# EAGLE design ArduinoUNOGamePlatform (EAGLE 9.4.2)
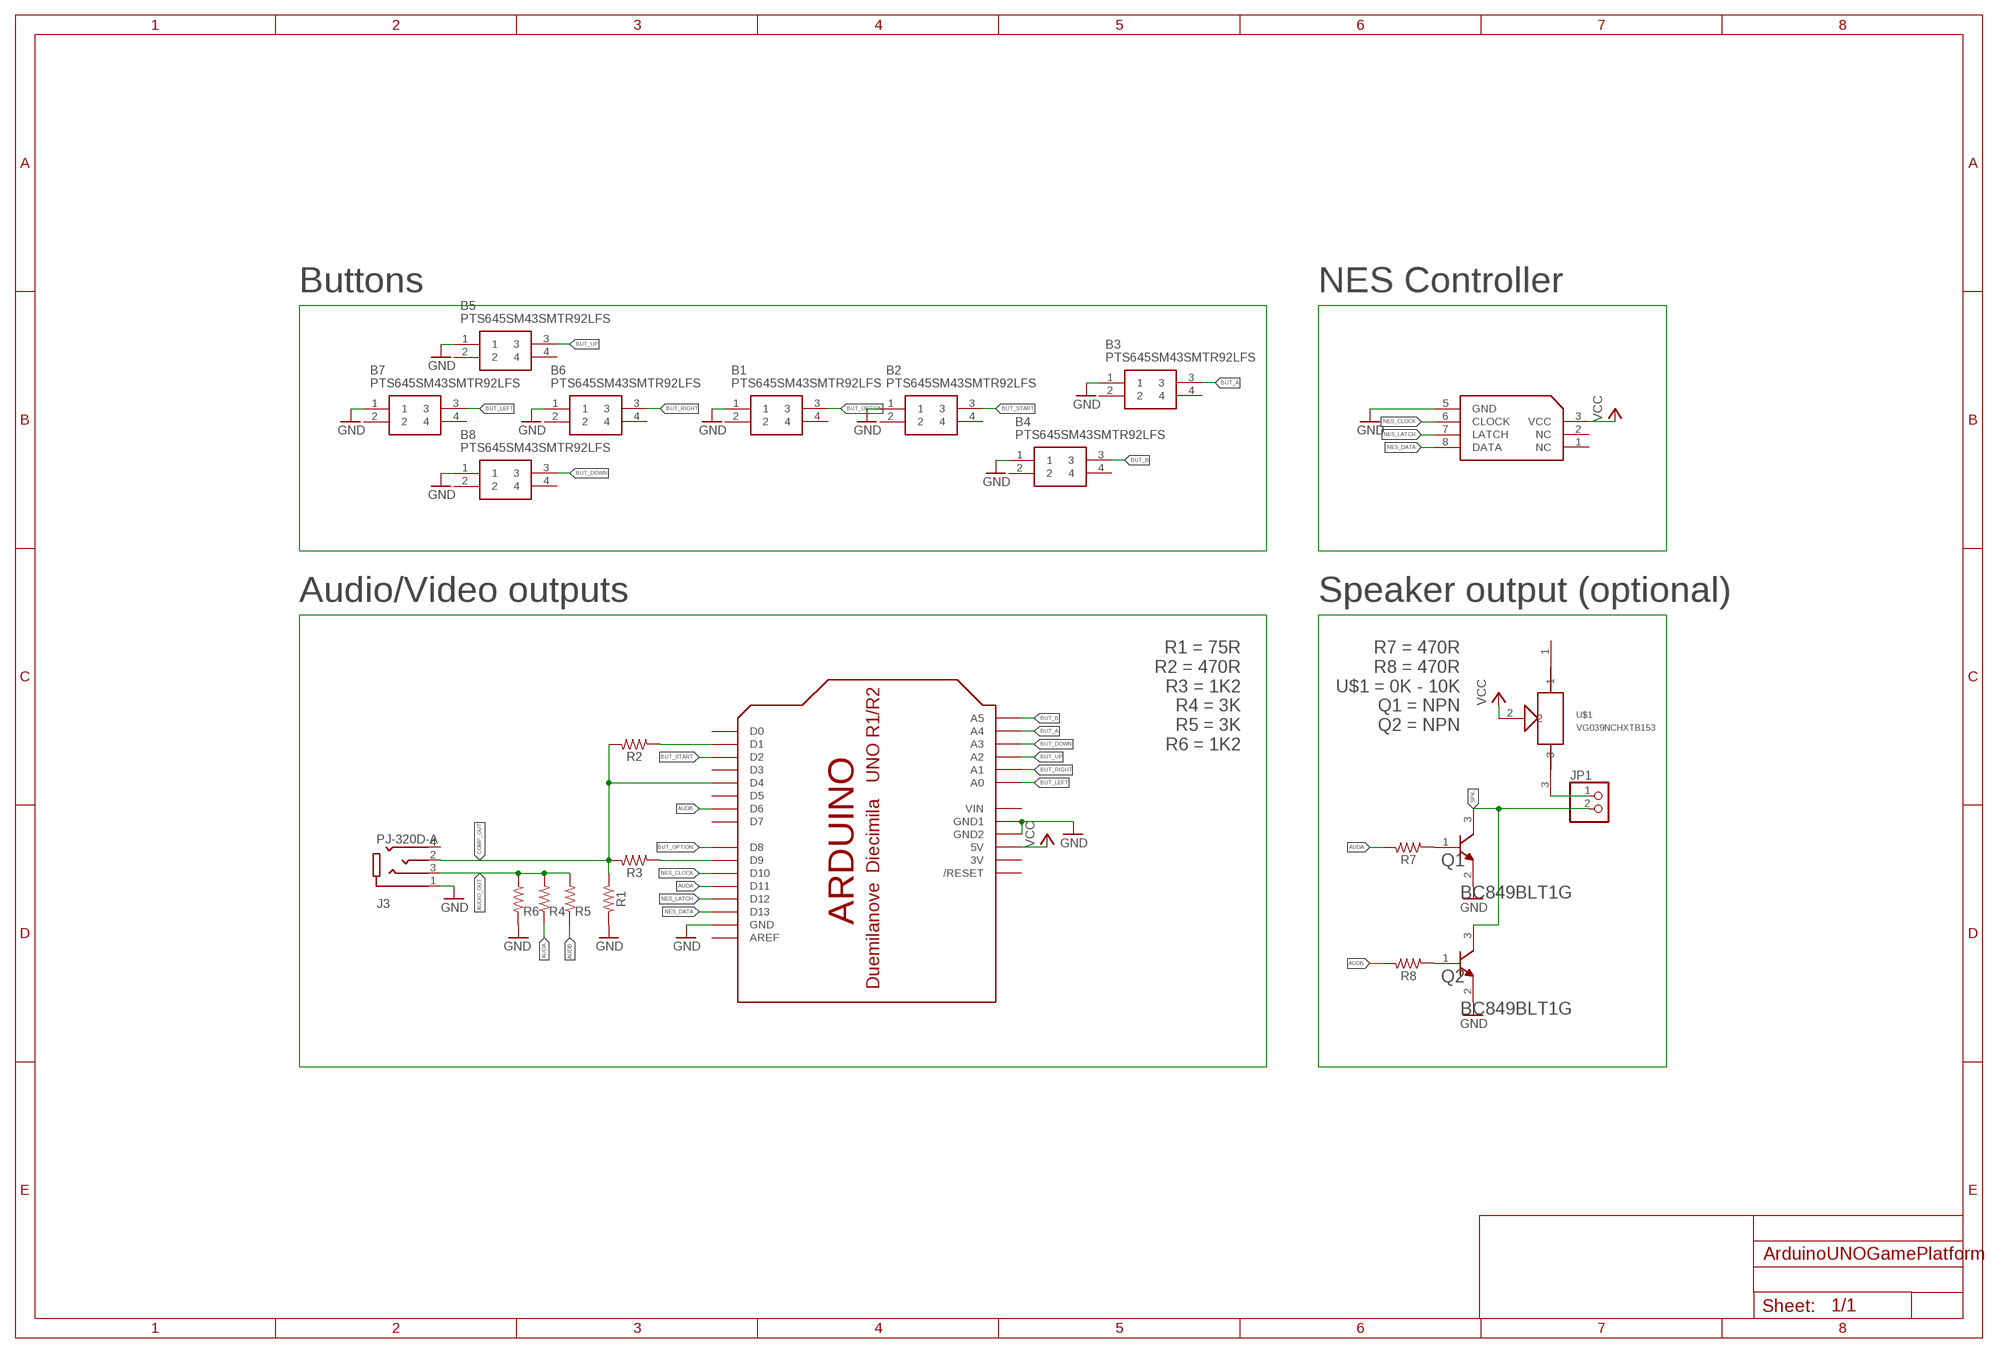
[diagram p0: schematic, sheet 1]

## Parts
B1  PTS645SM43SMTR92LFS  [PTS645(SMT)]
B2  PTS645SM43SMTR92LFS  [PTS645(SMT)]
B3  PTS645SM43SMTR92LFS  [PTS645(SMT)]
B4  PTS645SM43SMTR92LFS  [PTS645(SMT)]
B5  PTS645SM43SMTR92LFS  [PTS645(SMT)]
B6  PTS645SM43SMTR92LFS  [PTS645(SMT)]
B7  PTS645SM43SMTR92LFS  [PTS645(SMT)]
B8  PTS645SM43SMTR92LFS  [PTS645(SMT)]
J3  PJ-320D-A  [HRO_PJ-320D-A]
JP1  PINHD-1X2  [1X02]
Q1  ON_SEMICONDUCTOR_BC849BLT1GON_SEMICONDUCTOR_BC849BLT1G_0_0  [ON_SEMICONDUCTOR_BC849BLT1G_0]
Q2  ON_SEMICONDUCTOR_BC849BLT1GON_SEMICONDUCTOR_BC849BLT1G_0_0  [ON_SEMICONDUCTOR_BC849BLT1G_0]
R1  75R  52101-101-REV-A_RC-MASTER-SMD_R_0603MP  [52101-101-REV-A_RC-MASTER-SMD_R0603MP]
R2  220R  52101-101-REV-A_RC-MASTER-SMD_R_0603MP  [52101-101-REV-A_RC-MASTER-SMD_R0603MP]
R3  1K2  52101-101-REV-A_RC-MASTER-SMD_R_0603MP  [52101-101-REV-A_RC-MASTER-SMD_R0603MP]
R4  3K  52101-101-REV-A_RC-MASTER-SMD_R_0603MP  [52101-101-REV-A_RC-MASTER-SMD_R0603MP]
R5  3K  52101-101-REV-A_RC-MASTER-SMD_R_0603MP  [52101-101-REV-A_RC-MASTER-SMD_R0603MP]
R6  1K2  52101-101-REV-A_RC-MASTER-SMD_R_0603MP  [52101-101-REV-A_RC-MASTER-SMD_R0603MP]
R7  470R  52101-101-REV-A_RC-MASTER-SMD_R_0603MP  [52101-101-REV-A_RC-MASTER-SMD_R0603MP]
R8  470R  52101-101-REV-A_RC-MASTER-SMD_R_0603MP  [52101-101-REV-A_RC-MASTER-SMD_R0603MP]
U$1  VG039NCHXTB153  [VG039NCHXTB101]
U$2  ARDUINO-BPLACE  [ARDUINO-BPLACE]
U$3  NES-CONTROLLER-PORT  [NES-CONTROLLER-SOCKET]

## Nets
AUDA: R4.1 R7.2 U$2.D11
AUDB: R5.1 R8.2 U$2.D6
AUDIO_OUT: J3.3(RING1) R4.2 R5.2 R6.1
BUT_A: B3.3 U$2.A4
BUT_B: B4.3 U$2.A5
BUT_DOWN: B8.3 U$2.A3
BUT_LEFT: B7.3 U$2.A0
BUT_OPTION: B1.3 U$2.D8
BUT_RIGHT: B6.3 U$2.A1
BUT_START: B2.3 U$2.D2
BUT_UP: B5.3 U$2.A2
COMP_OUT: J3.2(TIP) R1.1 R2.2 R3.2 U$2.D4
GND: B1.1 B2.1 B3.1 B4.1 B5.1 B6.1 B7.1 B8.1 J3.1(SLEEVE) Q1.2(E) Q2.2(E) R1.2 R6.2 U$2.GND U$2.GND1 U$2.GND2 U$3.5(GND)
N$1: JP1.1 U$1.3
N$7: Q2.1(B) R8.1
N$8: Q1.1(B) R7.1
NES_CLOCK: U$2.D10 U$3.6(CLOCK)
NES_DATA: U$2.D13 U$3.8(DATA)
NES_LATCH: U$2.D12 U$3.7(LATCH)
SPK-: JP1.2 Q1.3(C) Q2.3(C)
SYNC_OUT: R3.1 U$2.D9
VCC: U$1.2 U$2.5V U$3.3(VCC)
VIDEO_OUT: R2.1 U$2.D1
Unconnected: B1.2 B1.4 B2.2 B2.4 B3.2 B3.4 B4.2 B4.4 B5.2 B5.4 B6.2 B6.4 B7.2 B7.4 B8.2 B8.4 J3.4(RING2) U$1.1 U$2.AREF U$2.D0 U$2.D3 U$2.D5 U$2.D7 U$2.RESET(/RESET) U$3.1(NC) U$3.2(NC)

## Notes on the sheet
- Buttons | NES Controller
- Audio/Video outputs | Speaker output (optional)
- R1 = 75R
  R2 = 470R
  R3 = 1K2
  R4 = 3K
  R5 = 3K
  R6 = 1K2
- R7 = 470R
  R8 = 470R
  U$1 = 0K - 10K
  Q1 = NPN
  Q2 = NPN

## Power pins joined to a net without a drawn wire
3V: U$2.3V
VIN: U$2.VIN

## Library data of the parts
B1-B8 = PTS645SM43SMTR92LFS:PTS645SM43SMTR92LFS: C & K COMPONENTS - PTS645SM43SMTR92LFS - SWITCH, SPST, 0.05A, 12VDC, SMD, 4.3MM Source: Datasheet; DESCRIPTION: C & K COMPONENTS - PTS645SM43SMTR92LFS - SWITCH, SPST, 0.05A, 12VDC, SMD, 4.3MM; HEIGHT: mm; MANUFACTURER_NAME: C & K COMPONENTS; MANUFACTURER_PART_NUMBER: PTS645SM43SMTR92LFS; MOUSER_PART_NUMBER: 611-PTS645SM43SMTR92; MOUSER_PRICE-STOCK: https://www.mouser.com/Search/Refine.aspx?Keyword=611-PTS645SM43SMTR92
J3 = PJ-320D-A:PJ-320D-A: Check availability; AVAILABILITY: Not in stock; CHECK_PRICES: https://www.snapeda.com/parts/PJ-320D-A/HRO+Electronics+Co.%252C+Ltd./view-part/?ref=eda; DESCRIPTION: Headphone jack 0.5A 30V DC 100 mΩ; MF: HRO Electronics Co., Ltd.; MP: PJ-320D-A; PACKAGE: Package; PRICE: None; SNAPEDA_LINK: https://www.snapeda.com/parts/PJ-320D-A/HRO+Electronics+Co.%252C+Ltd./view-part/?ref=snap
JP1 = pinhead:PINHD-1X2: PIN HEADER
Q1 Q2 = On Semiconductor - BC849BLT1G:ON_SEMICONDUCTOR_BC849BLT1G: ONSC-NPN-B1E2C3-3; CIIVA_IDS: 19369299; COMPONENT_LINK_1_DESCRIPTION: Manufacturer URL; COMPONENT_LINK_1_URL: http://www.onsemi.com/; COMPONENT_LINK_3_DESCRIPTION: Package Specification; COMPONENT_LINK_3_URL: http://www.onsemi.cn/pub_link/Collateral/318-08.PDF; DATASHEET: http://www.onsemi.cn/pub_link/Collateral/BC846ALT1-D.PDF; DATASHEET_VERSION: Rev. 11; FOOTPRINT_VARIANT_NAME_0: Manufacturer Recommended; FT_MIN_MHZ: 100; IC_CONTINUOUS_A: 0.1; IMPORTED: yes; IMPORTED_FROM: vault; IMPORT_TS: 1521843736; MF: On Semiconductor; MOUNTING_TECHNOLOGY: Surface Mount; MPN: BC849BLT1G; PACKAGE: SOT-23-3-318-08; PACKAGE_DESCRIPTION: 3-Pin Small Outline Transistor, Body 2.92 x 1.3 mm, Pitch 0.95 mm; PACKAGE_VERSION: Rev. AP, 11/2009; PACKING: Tape and Reel; POLARITY: NPN; PREFIX: Q; RELEASE_DATE: 1406898388; ROHS: Yes; VAULT_GUID: 19D3C7D6-08FD-4A81-9BD4-62C7617130FB; VAULT_REVISION: B4675A61-FAF7-4072-9C56-0A9635A35669
R1-R8 = ESP32_DMX_Audio:52101-101-REV-A_RC-MASTER-SMD_R_: RESISTOR
U$1 = untitled:VG039NCHXTB153
U$2 = adafruit:ARDUINO: Arduino Diecimila/Duemilanove Make a shield with ease, this package has all the named pins as well as the two mounting drill holes and an outline of the USB and DC power connector. The outline is on the DIMENSION layer, so if your board house uses it they will cut the outline to match.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
U$3 = PJ-320D-A:NES-CONTROLLER-PORT

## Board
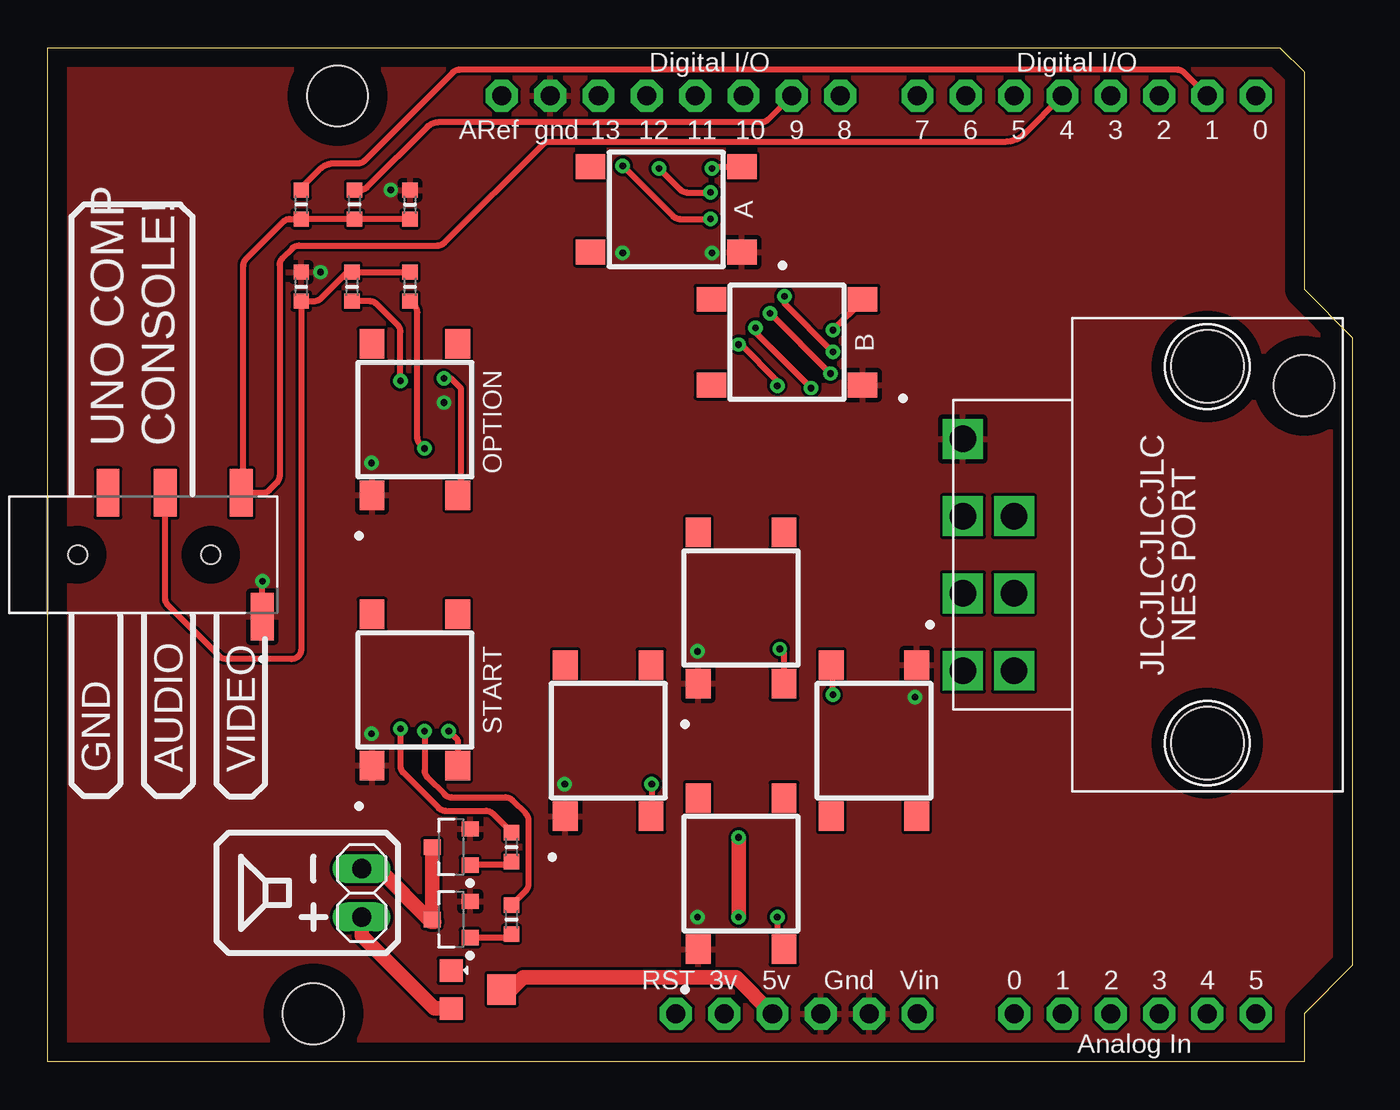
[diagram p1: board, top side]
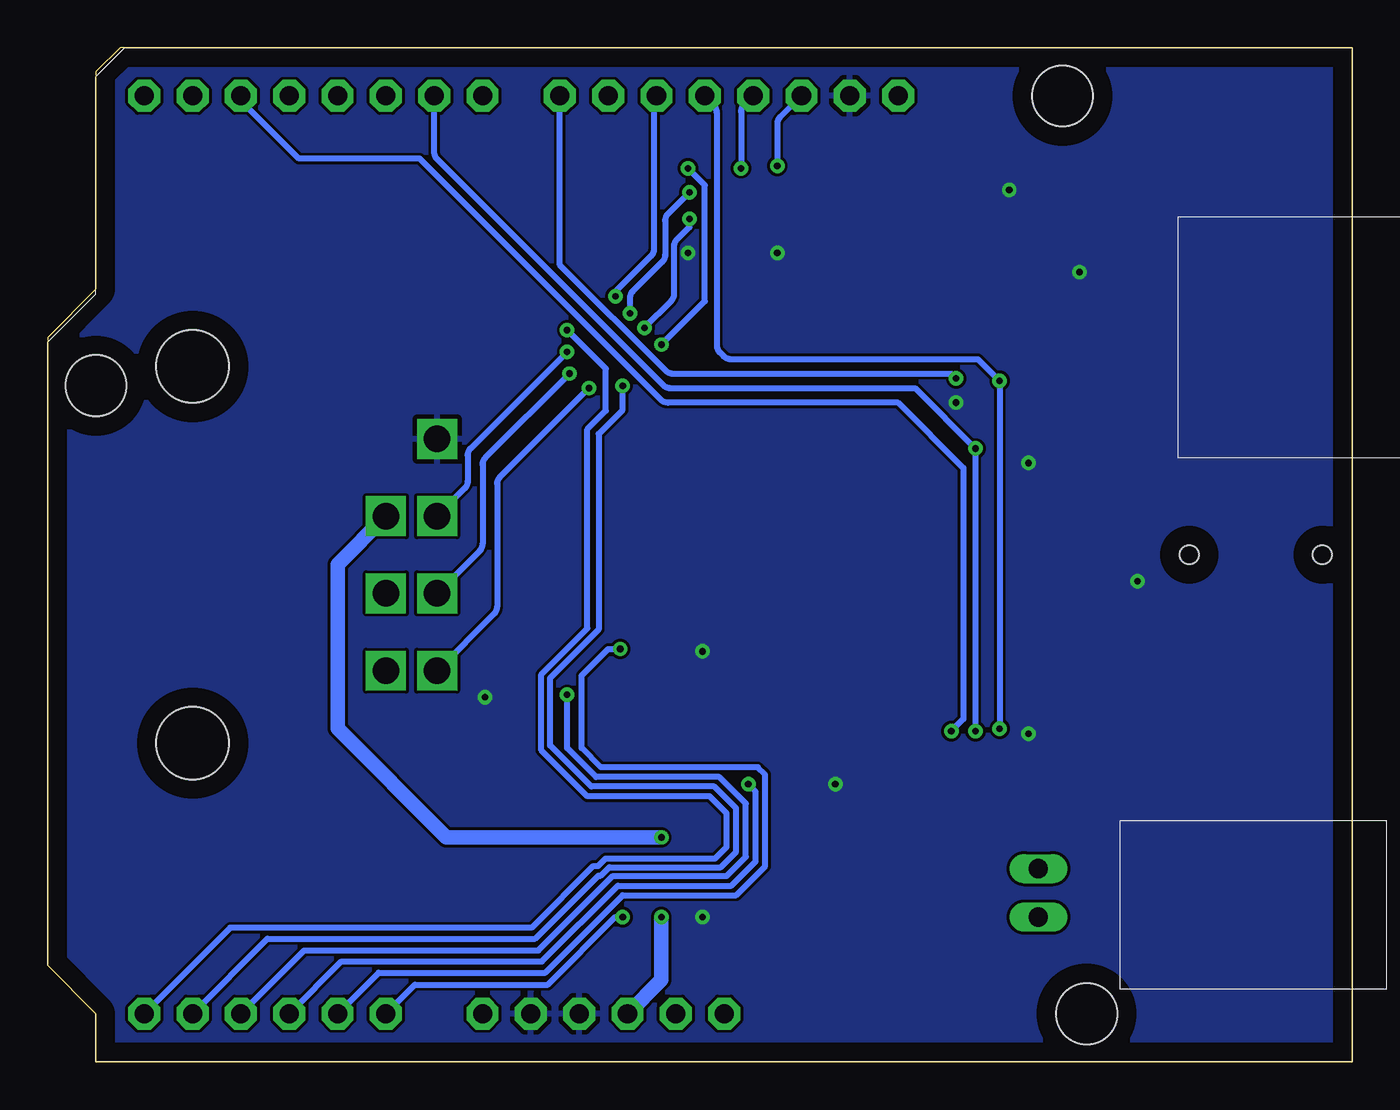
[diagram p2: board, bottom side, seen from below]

Size 68.58 x 53.34 mm. Coordinates in mm from the lower left corner, seen from the top.
Outline: 0,53.34 64.77,53.34 66.04,52.07 66.04,40.64 68.58,38.1 68.58,5.08 66.04,2.54 66.04,0 0,0 0,53.34
Copper layers (1*16): Top 0.035mm / dielectric 0.15mm / Bottom 0.035mm
Design rules "default": minimum track width 6mil, minimum drill 0.35mm, track to track 6mil, track to pad 6mil, pad to pad 6mil, via to via 6mil, smd to smd 6mil, copper to edge 40mil, drill to drill 6mil, minimum pad ring 10mil, minimum via ring 8mil, stop-mask expansion 4mil, vias tented up to drill 0mil, thermal gap 10mil

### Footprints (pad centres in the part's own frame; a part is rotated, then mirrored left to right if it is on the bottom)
PTS645(SMT) = smd 1.55 x 1.3: 1 -3.975,2.25; 2 3.975,2.25; 3 -3.975,-2.25; 4 3.975,-2.25
HRO_PJ-320D-A = smd 1.2 x 2.5: 1 6.2,-3.25; 2 5.1,3.25; 3 1.1,3.25; 4 -1.9,3.25 | hole 1: -3.5,0; 3.5,0
1X02 = drill 1.016 long: 1 -1.27,0; 2 1.27,0
ON_SEMICONDUCTOR_BC849BLT1G_0 = smd 0.9 x 0.8: 1 -1,0.95; 2 -1,-0.95; 3 1,0
52101-101-REV-A_RC-MASTER-SMD_R0603MP = smd 0.8 x 0.8: 1 -0.762,0; 2 0.762,0
VG039NCHXTB101 = smd 1.2 x 1.2: 1 -1,-1.65; 3 1,-1.65 | smd 1.6 x 1.5: 2 0,1
ARDUINO-BPLACE = drill 1 pad 1.676 octagon: 3V 35.56,2.54; 5V 38.1,2.54; A0 50.8,2.54; A1 53.34,2.54; A2 55.88,2.54; A3 58.42,2.54; A4 60.96,2.54; A5 63.5,2.54; AREF 23.876,50.8; D0 63.5,50.8; D1 60.96,50.8; D2 58.42,50.8; D3 55.88,50.8; D4 53.34,50.8; D5 50.8,50.8; D6 48.26,50.8; D7 45.72,50.8; D8 41.656,50.8; D9 39.116,50.8; D10 36.576,50.8; D11 34.036,50.8; D12 31.496,50.8; D13 28.956,50.8; GND 26.416,50.8; GND1 43.18,2.54; GND2 40.64,2.54; RESET 33.02,2.54; VIN 45.72,2.54 | hole 3.2: 15.24,50.8; 66.04,35.56; 13.97,2.54
NES-CONTROLLER-SOCKET = drill 1.4 square: 1 6.096,-10.16; 2 2.032,-10.16; 3 -2.032,-10.16; 5 -6.096,-12.852; 6 -2.032,-12.852; 7 2.032,-12.852; 8 6.096,-12.852 | hole 3.8: -9.906,0; 9.906,0

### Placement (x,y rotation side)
B1  19.3,33.78 90 top
B2  19.3,19.56 90 top
B3  32.51,44.83 180 top
B4  38.86,37.85 180 top
B5  29.46,16.89 90 top
B6  36.45,23.88 90 top
B7  36.45,9.91 90 top
B8  43.43,16.89 270 top
J3  5.08,26.67 0 top
JP1  16.51,8.89 90 top
Q1  21.21,11.3 180 top
Q2  21.21,7.49 180 top
R1  19.05,45.09 90 top
R2  13.34,45.09 270 top
R3  16.13,45.09 270 top
R4  16,40.77 90 top
R5  19.05,40.77 90 top
R6  13.34,40.77 90 top
R7  24.38,11.3 90 top
R8  24.38,7.49 90 top
U$1  22.86,3.81 270 top
U$2  0,0 0 top
U$3  60.96,26.67 270 top

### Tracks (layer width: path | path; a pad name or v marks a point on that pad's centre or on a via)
AUDA  (via drill 0.35)
  Top 0.305: R7.2 23.39,13.06 arc45 23.03,13.21 20.91,13.21 arc-45 20.55,13.36 18.69,15.22 arc-45 18.54,15.58 v18.54,17.53 | v18.54,35.81 18.54,38.4 arc45 18.39,38.76 17.29,39.86 arc45 16.93,40.01 R4.1
  Bottom 0.305: U$2.D11 33.68,50.44 arc45 33.4,49.77 33.4,37.67 arc-45 33.25,37.32 33.04,37.11 arc-45 32.68,36.96 19.68,36.96 v18.54,35.81 v18.54,17.53
AUDB  (via drill 0.35)
  Top 0.305: R8.2 25.12,8.99 arc45 25.27,9.35 25.27,12.71 arc45 25.12,13.06 24.42,13.76 arc45 24.07,13.91 21.22,13.91 arc-45 20.86,14.06 19.96,14.96 arc-45 19.81,15.32 v19.81,17.4 | v19.81,32.26 19.58,32.49 arc-45 19.43,32.85 19.43,39.41 arc45 19.28,39.77 R5.1
  Bottom 0.305: U$2.D6 48.26,47.84 arc-45 48.11,47.48 36.22,35.58 arc-45 35.86,35.43 22.99,35.43 v19.81,32.26 v19.81,17.4
AUDIO_OUT
  Top 0.305: J3.3 6.18,24.38 arc45 6.33,24.02 9.01,21.34 arc45 9.37,21.19 12.83,21.19 arc90 13.34,21.7 R6.1 14.01,40.01 arc45 14.37,40.15 15.75,41.53 R4.2 R5.2
BUT_A  (via drill 0.35)
  Top 0.305: v38.35,35.56 38.35,35.81 36.45,37.72 v36.32,37.72 | v34.92,46.99 35.02,47.08 B3.3
  Bottom 0.305: U$2.A4 57.02,6.48 42.95,6.48 39.64,9.79 39.51,9.79 39.06,10.24 33.19,10.24 32.38,11.05 32.38,13.34 33.53,14.48 40.01,14.48 42.16,16.64 42.16,20.19 39.62,22.73 39.62,33.02 38.35,34.29 v38.35,35.56 | v34.92,46.99 34.04,46.1 34.04,40.01 v36.32,37.72
BUT_B  (via drill 0.35)
  Top 0.305: B4.3 42.84,40.04 v41.27,38.48
  Bottom 0.305: U$2.A5 58.98,7.06 43.14,7.06 39.9,10.3 39.64,10.3 39.25,10.7 33.5,10.7 32.89,11.3 32.89,13.08 33.78,13.97 40.21,13.97 42.62,16.38 42.62,20.38 40.21,22.8 40.21,33.27 39.24,34.24 39.24,36.45 v41.27,38.48
BUT_DOWN  (via drill 0.35)
  Top 0.305: v41.27,19.3 41.27,20.77 B8.3
  Bottom 0.305: U$2.A3 55.09,5.87 42.78,5.87 38.87,9.79 32.89,9.79 31.88,10.79 31.88,13.59 33.27,14.99 39.75,14.99 41.27,16.51 v41.27,19.3
BUT_LEFT  (via drill 0.35)
  Top 0.305: v38.35,7.62 38.35,6.28 B7.3
  Bottom 0.305: U$2.A0 49.28,4.06 42.29,4.06 38.73,7.62 v38.35,7.62
BUT_OPTION  (via drill 0.35)
  Top 0.305: v20.83,35.94 21.21,35.94 21.72,35.43 21.72,29.97 B1.3
  Bottom 0.305: v20.83,35.94 21.08,36.2 35.73,36.2 arc45 36.09,36.34 41.66,41.91 U$2.D8
BUT_RIGHT  (via drill 0.35)
  Top 0.305: v38.48,21.72 38.7,21.5 B6.3
  Bottom 0.305: U$2.A1 51.18,4.7 42.42,4.7 38.35,8.76 32.38,8.76 30.86,10.29 30.86,15.11 31.24,15.49 39.5,15.49 40.51,16.51 40.51,20.32 39.12,21.72 v38.48,21.72
BUT_START  (via drill 0.35)
  Top 0.305: v21.08,17.4 21.55,16.93 B2.3
  Bottom 0.305: U$2.D2 58.42,50.55 55.37,47.5 49.02,47.5 36.34,34.82 arc-45 35.98,34.67 23.88,34.67 20.45,31.24 20.45,18.03 v21.08,17.4
BUT_UP  (via drill 0.35)
  Top 0.305: v31.75,14.61 31.75,12.95 B5.3
  Bottom 0.305: U$2.A2 53.14,5.28 42.6,5.28 38.61,9.27 32.64,9.27 31.37,10.54 31.37,14.22 v31.75,14.61
COMP_OUT
  Top 0.305: R1.1 R3.2 R2.2 12.74,44.32 arc45 12.38,44.17 10.44,42.23 arc45 10.29,41.87 10.29,30.03 J3.2 11.29,29.92 arc45 11.65,30.07 12.04,30.46 arc45 12.19,30.82 12.19,41.9 arc-45 12.34,42.26 12.86,42.78 arc-45 13.21,42.93 20.49,42.93 arc45 20.85,43.08 26.01,48.24 arc-45 26.37,48.39 50.36,48.39 arc45 51.33,48.79 U$2.D4
GND  (via drill 0.35)
  Top 0.305: J3.1 11.28,25.25 v11.3,25.27
  other vias: 17.02,31.5 20.83,34.67 18.03,45.85 34.92,42.55 17.02,17.27 34.16,21.59 27.18,14.61 45.59,19.18 34.16,7.62 14.35,41.53 30.23,42.55
  pour Bottom: -2.54,54.61 72.39,54.61 72.39,-3.81 -2.54,-3.81
  pour Top: -2.54,54.61 72.39,54.61 72.39,-3.81 -2.54,-3.81
N$1
  Top 0.762: U$1.3 20.32,2.81 16.51,6.62 JP1.1
N$7
  Top 0.305: Q2.1 24.2,6.54 R8.1
N$8
  Top 0.305: R7.1 24.2,10.35 Q1.1
NES_CLOCK  (via drill 0.35)
  Top 0.305: v38.73,40.26 38.73,39.88 v41.27,37.34
  Bottom 0.305: U$2.D10 36.7,50.67 36.7,42.76 arc45 36.85,42.4 38.73,40.51 v38.73,40.26 | U$3.6 46.65,30.17 arc-45 46.5,30.53 46.5,31.9 arc45 46.35,32.26 v41.27,37.34
NES_DATA  (via drill 0.35)
  Top 0.305: v30.23,47.12 32.87,44.47 arc45 33.23,44.32 v34.85,44.32 | v40.13,35.43 37.21,38.35 v37.21,38.61
  Bottom 0.305: U$2.D13 30.08,49.68 arc-45 30.23,49.32 v30.23,47.12 | v34.85,44.32 34.85,43.89 35.51,43.23 arc-45 35.66,42.87 35.66,40.37 arc45 35.81,40.01 v37.21,38.61 | v40.13,35.43 44.81,30.76 arc-45 44.96,30.4 44.96,23.93 arc45 45.11,23.57 U$3.8
NES_LATCH  (via drill 0.35)
  Top 0.305: v32.13,46.99 33.25,45.87 arc45 33.61,45.72 v34.85,45.72 | v37.97,39.37 v41.15,36.2
  Bottom 0.305: U$2.D12 31.98,50.31 arc-45 32.13,49.95 v32.13,46.99 | v34.85,45.72 35.97,44.6 arc-45 36.12,44.24 36.12,42.44 arc45 36.27,42.08 37.82,40.52 arc-45 37.97,40.16 v37.97,39.37 | v41.15,36.2 45.57,31.77 arc-45 45.72,31.41 45.72,27.24 arc45 45.87,26.88 U$3.7
SPK-
  Top 0.508: 20.32,7.38 Q2.3
  Top 0.762: Q1.3 Q2.3 | 20.32,7.38 20.18,7.38 17.4,10.16 JP1.2
SYNC_OUT
  Top 0.305: R3.1 16.43,45.85 arc45 16.79,46 19.95,49.16 arc-45 20.53,49.4 37.51,49.4 arc45 37.87,49.55 U$2.D9
VCC  (via drill 0.35)
  Top 0.762: U$2.5V 36.2,4.45 25,4.45 24.37,3.81 U$1.2 | v36.32,7.62 v36.32,11.81
  Bottom 0.762: U$2.5V 36.32,4.32 v36.32,7.62 | v36.32,11.81 47.62,11.81 53.34,17.53 53.34,26.16 U$3.3
VIDEO_OUT
  Top 0.305: R2.1 13.34,45.97 14.28,46.92 arc-45 15.07,47.24 16.3,47.24 arc45 16.66,47.39 21.29,52.02 arc-45 21.65,52.17 59.38,52.17 arc-45 59.74,52.02 U$2.D1

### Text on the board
tPlace: A | B | OPTION | UNO COMP / CONSOLE! | JLCJLCJLCJLC | START | GND | AUDIO | VIDEO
